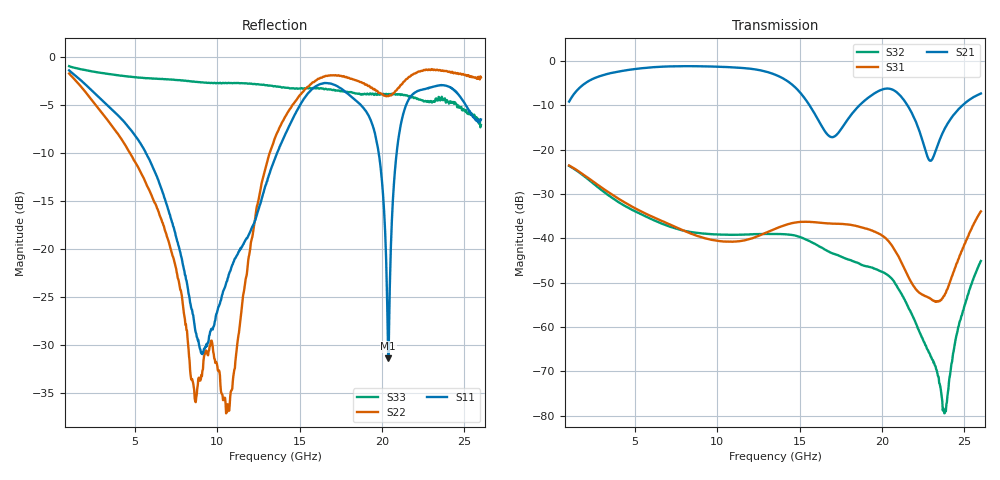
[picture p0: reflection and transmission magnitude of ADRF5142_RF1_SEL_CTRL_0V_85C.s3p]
! Device: ADRF5142
! Description: Silicon, SPDT Switch, Reflective
! Frequency: 8.00 GHz - 11.00 GHz
! Ports:
!  RFC = Port 1
!  RF1 = Port 2
!  RF2 = Port 3
! VDD = +3.3V
! VSS = -3.3V
! CTRL = 0V
! Temp = 85C
! Data:  Data was collected using an calibrated 4 port network analyzer.
!  The reference plane is the package pins of ADRF5142 switch.
! Notes: Analog Devices supplies this data as a sample of measured data
!  for this product.  Your particular data for this product may vary.
!  Data was taken at 85 degrees C.
!  Analog Devices reserves the right to change this data at anytime.
# HZ S DB R 50
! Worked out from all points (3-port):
!   801 points, 1 GHz to 26 GHz, reference 50 ohm
!   strongest paths, dB at 1 GHz, 7.25 GHz, 13.5 GHz, 19.75 GHz, 26 GHz:
!     S21: -9.1, -1.2, -3.0, -6.8, -7.3
!     S31: -23.5, -37.1, -37.9, -38.8, -33.9
!     S32: -23.6, -37.5, -39.0, -47.1, -45.1
!   lowest |S11| = -31.4 dB at 20.38 GHz (marker M1), VSWR 1.06, Z = 48.7 + j2.29 ohm
!   |S11| at or under -10 dB: 5.655 GHz to 13.63 GHz (7.973 GHz wide, 82.7 % of centre); 19.8 GHz to 20.88 GHz (1.088 GHz wide, 5.35 % of centre)
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1e9  -1.39 158.2  -9.12 36.4  -23.55 -37.5
     -9.12 36.4  -1.72 125.3  -23.63 -55.0
     -23.55 -37.5  -23.63 -55.0  -0.95 171.0
2.9687e9  -4.44 128.2  -3.25 -18.5  -28.51 -86.9
          -3.25 -18.5  -5.75 35.6  -29.11 -138.9
          -28.51 -86.9  -29.11 -138.9  -1.66 157.6
6.2187e9  -12.01 91.0  -1.33 -94.1  -35.39 -128.2
          -1.33 -94.1  -15.24 -80.3  -36.02 130.2
          -35.39 -128.2  -36.02 130.2  -2.26 139.5
1.0625e10  -23.07 -155.4  -1.33 166.9  -40.73 -154.9
           -1.33 166.9  -36.19 126.6  -39.16 33.7
           -40.73 -154.9  -39.16 33.7  -2.71 112.4
1.35e10  -10.56 -117.3  -3.03 91.9  -37.86 -173.7
         -3.03 91.9  -8.42 69.0  -39.00 -38.5
         -37.86 -173.7  -39.00 -38.5  -3.03 95.5
1.89375e10  -5.47 91.5  -8.91 63.2  -37.70 78.4
            -8.91 63.2  -2.81 -88.6  -46.18 146.8
            -37.70 78.4  -46.18 146.8  -3.82 55.3
2.0375e10  -31.40 119.2  -6.18 12.6  -40.54 42.0
           -6.18 12.6  -4.08 -107.0  -48.35 86.9
           -40.54 42.0  -48.35 86.9  -3.86 42.6
2.12812e10  -5.96 177.7  -8.53 -27.8  -46.21 26.5
            -8.53 -27.8  -2.64 -112.4  -53.20 44.3
            -46.21 26.5  -53.20 44.3  -3.95 36.9
2.38125e10  -2.96 65.1  -15.17 20.9  -52.65 131.8
            -15.17 20.9  -1.46 -162.8  -79.44 -77.2
            -52.65 131.8  -79.44 -77.2  -4.31 8.8
2.6e10  -6.51 -40.7  -7.29 -28.2  -33.91 138.6
        -7.29 -28.2  -2.13 165.7  -45.11 147.0
        -33.91 138.6  -45.11 147.0  -7.10 -12.4
